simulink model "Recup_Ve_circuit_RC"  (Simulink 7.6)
settings: Solver=ode15s  StartTime=0.0  StopTime=10.0  RelTol=1e-3
InitFcn:
  | R=1e3;
  | C=1e-3;
  | U0=5;
StopFcn:
  | load circuit_RC.mat
  | plotyy(y(1,:),y(2,:),y(1,:),y(3,:))
  | title('Tension aux bornes de C, courant dans le circuit RC')
  | grid
  | axis([0 10 -0.5 5.5])
libraries: fl_lib x12, nesl_utility x5, elec_lib x1

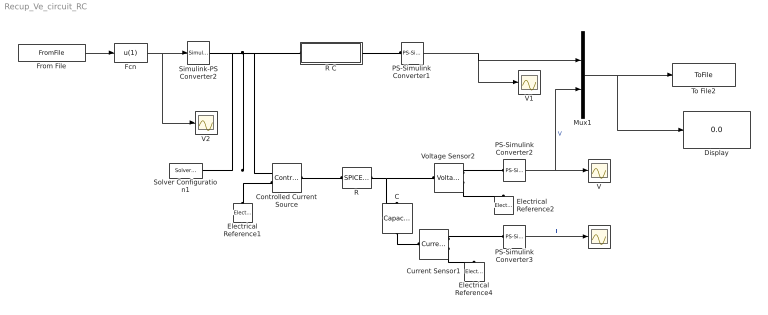
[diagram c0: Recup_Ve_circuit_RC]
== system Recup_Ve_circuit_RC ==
  C : fl_lib/Electrical/Electrical Elements/Capacitor  DialogController=NetworkEngine.DynNeDlgSource  SystemSampleTime=-1  c=C F  v0=0 V  r=1e-06 Ohm  g=0 1/Ohm  i_Log=off  v_Log=off  vc_Log=off  LocalVarNames=|i|v|vc  LocalVarDescs=|i|v|Internal variable for voltage across capacitor term  LocalVarLogging=[0 0 0]
  Controlled Current Source : fl_lib/Electrical/Electrical Sources/Controlled Current Source  DialogController=NetworkEngine.DynNeDlgSource  SystemSampleTime=-1  i_Log=off  v_Log=off  LocalVarNames=|i|v  LocalVarDescs=|i|v  LocalVarLogging=[0 0]
  Current Sensor1 : fl_lib/Electrical/Electrical Sensors/Current Sensor  DialogController=NetworkEngine.DynNeDlgSource  SystemSampleTime=-1  i1_Log=off  v1_Log=off  LocalVarNames=|i1|v1  LocalVarDescs=|i1|v1  LocalVarLogging=[0 0]
  Display : Display
  Electrical Reference1 : fl_lib/Electrical/Electrical Elements/Electrical Reference  DialogController=NetworkEngine.DynNeDlgSource  SystemSampleTime=-1  i_Log=off  LocalVarNames=|i  LocalVarDescs=|i  LocalVarLogging=[]
  Electrical Reference2 : fl_lib/Electrical/Electrical Elements/Electrical Reference  DialogController=NetworkEngine.DynNeDlgSource  SystemSampleTime=-1  i_Log=off  LocalVarNames=|i  LocalVarDescs=|i  LocalVarLogging=[]
  Electrical Reference4 : fl_lib/Electrical/Electrical Elements/Electrical Reference  DialogController=NetworkEngine.DynNeDlgSource  SystemSampleTime=-1  i_Log=off  LocalVarNames=|i  LocalVarDescs=|i  LocalVarLogging=[]
  Fcn : Fcn  Expr=u(1)
  From File : FromFile  FileName=appli_circuit_RC  SampleTime=0
  I : Scope
  Mux1 : Mux  Inputs=2
  PS-Simulink Converter1 : nesl_utility/PS-Simulink Converter  DialogController=NetworkEngine.DynNeUtilDlgSource  SystemSampleTime=-1  PhysicalDomain=network_engine_domain  LeftPortType=input  RightPortType=output  SubClassName=ps_output  Unit=1  AffineConversion=off
  PS-Simulink Converter2 : nesl_utility/PS-Simulink Converter  DialogController=NetworkEngine.DynNeUtilDlgSource  SystemSampleTime=-1  PhysicalDomain=network_engine_domain  LeftPortType=input  RightPortType=output  SubClassName=ps_output  Unit=1  AffineConversion=off
  PS-Simulink Converter3 : nesl_utility/PS-Simulink Converter  DialogController=NetworkEngine.DynNeUtilDlgSource  SystemSampleTime=-1  PhysicalDomain=network_engine_domain  LeftPortType=input  RightPortType=output  SubClassName=ps_output  Unit=1  AffineConversion=off
  R : elec_lib/Additional Components/SPICE-Compatible Components/Passive Devices/SPICE Resistor  DialogController=NetworkEngine.DynNeDlgSource  SystemSampleTime=-1  SCALE=1  R_param=1  R=R Ohm  RSH=0 Ohm  LENGTH=1e-06 m  WIDTH=1e-06 m  NARROW=0 m  T_param=1  TC1=0 1/K  TC2=0 1/K^2  TOFFSET=0 K  TFIXED=300.15 K  TMEAS=300.15 K  LocalVarLogging=[]
  R C : Subsystem
  Simulink-PS Converter2 : nesl_utility/Simulink-PS Converter  DialogController=NetworkEngine.DynNeUtilDlgSource  SystemSampleTime=-1  PhysicalDomain=network_engine_domain  LeftPortType=input  RightPortType=output  SubClassName=ps_input  Unit=1  AffineConversion=off  InputFilterTimeConstant=.001  UdotUserProvided=0
  Solver Configuration1 : nesl_utility/Solver Configuration  DialogController=NetworkEngine.DynNeUtilDlgSource  SystemSampleTime=-1  PhysicalDomain=network_engine_domain  LeftPortType=input  RightPortType=generic  SubClassName=solver  Accelerate=off  Profile=off  ResidualTolerance=1e-9  MaxNonlinIter=12  MaxModeIter=2  DoFixedCost=off  UseLocalSampling=off  DoDC=off  LinearAlgebra=Sparse  LocalSolverSampleTime=.001  LocalSolverChoice=NE_BACKWARD_EULER_ADVANCER  UseLocalSolver=off
  To File2 : ToFile  Filename=circuit_RC.mat  MatrixName=y
  V : Scope
  V1 : Scope
  V2 : Scope
  Voltage Sensor2 : fl_lib/Electrical/Electrical Sensors/Voltage Sensor  DialogController=NetworkEngine.DynNeDlgSource  SystemSampleTime=-1  i1_Log=off  v1_Log=off  LocalVarNames=|i1|v1  LocalVarDescs=|i1|v1  LocalVarLogging=[]
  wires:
  From File/1 -> Fcn/1
  Fcn/1 -> Simulink-PS Converter2/1, V2/1
  PS-Simulink Converter2/1 -> V/1, Mux1/2  "V"
  PS-Simulink Converter1/1 -> Mux1/1, V1/1
  Mux1/1 -> To File2/1, Display/1
  PS-Simulink Converter3/1 -> I/1  "I"
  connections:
  Controlled Current Source/RConn1 -- Solver Configuration1/RConn1 -- Simulink-PS Converter2/RConn1 -- R C/LConn1
  R C/RConn1 -- PS-Simulink Converter1/LConn1
  R/RConn1 -- C/LConn1 -- Voltage Sensor2/LConn1
  R/LConn1 -- Controlled Current Source/LConn1
  Electrical Reference1/LConn1 -- Controlled Current Source/RConn2
  Voltage Sensor2/RConn1 -- PS-Simulink Converter2/LConn1
  Voltage Sensor2/RConn2 -- Electrical Reference2/LConn1
  C/RConn1 -- Current Sensor1/LConn1
  Current Sensor1/RConn2 -- Electrical Reference4/LConn1
  Current Sensor1/RConn1 -- PS-Simulink Converter3/LConn1

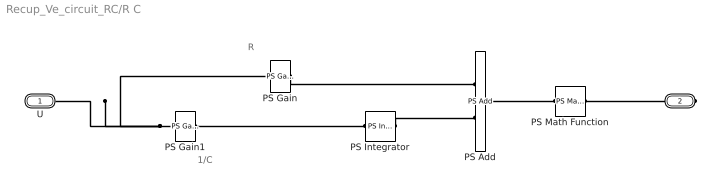
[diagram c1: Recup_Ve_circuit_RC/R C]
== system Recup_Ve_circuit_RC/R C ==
  note: 1/C
  note: R
  PS Add : fl_lib/Physical Signals/Functions/PS Add  DialogController=NetworkEngine.DynNeDlgSource  SystemSampleTime=-1  LocalVarLogging=[]
  PS Gain : fl_lib/Physical Signals/Functions/PS Gain  DialogController=NetworkEngine.DynNeDlgSource  SystemSampleTime=-1  gain=R  LocalVarLogging=[]
  PS Gain1 : fl_lib/Physical Signals/Functions/PS Gain  DialogController=NetworkEngine.DynNeDlgSource  SystemSampleTime=-1  gain=1/C  LocalVarLogging=[]
  PS Integrator : fl_lib/Physical Signals/Linear Operators/PS Integrator  DialogController=NetworkEngine.DynNeDlgSource  SystemSampleTime=-1  x0=0  x_Log=off  LocalVarNames=|x  LocalVarDescs=|x  LocalVarLogging=0
  PS Math Function : fl_lib/Physical Signals/Functions/PS Math Function  DialogController=NetworkEngine.DynNeDlgSource  SystemSampleTime=-1  fcn_choice=9  LocalVarLogging=[]
  U : PMIOPort  Port=1  Side=Left
  I : PMIOPort  Port=2  Side=Right
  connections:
  PS Gain1/LConn1 -- PS Gain/LConn1 -- U/RConn1
  PS Gain/RConn1 -- PS Add/LConn1
  PS Gain1/RConn1 -- PS Integrator/LConn1
  PS Integrator/RConn1 -- PS Add/LConn2
  PS Math Function/RConn1 -- I/RConn1
  PS Add/RConn1 -- PS Math Function/LConn1
